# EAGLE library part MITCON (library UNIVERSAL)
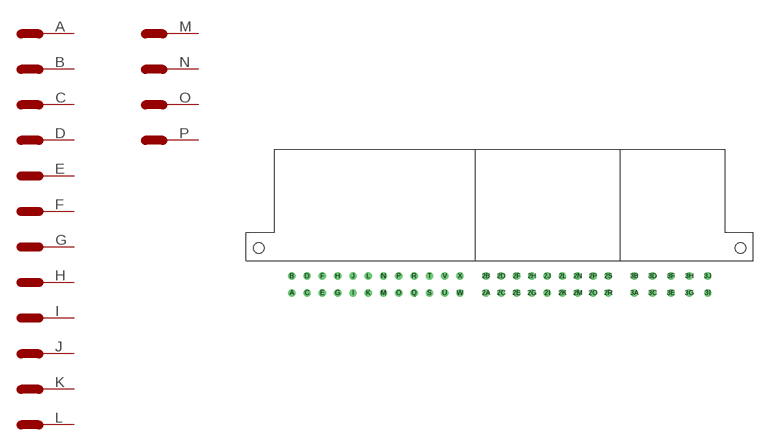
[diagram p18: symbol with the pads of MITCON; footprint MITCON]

Designator prefix CON; gates A=PIN B=PIN C=PIN D=PIN E=PIN F=PIN G=PIN H=PIN I=PIN J=PIN K=PIN L=PIN M=PIN N=PIN O=PIN P=PIN Q=PIN R=PIN S=PIN T=PIN U=PIN V=PIN W=PIN X=PIN 2A=PIN 2B=PIN 2C=PIN 2D=PIN 2E=PIN 2F=PIN 2G=PIN 2H=PIN 2I=PIN 2J=PIN 2K=PIN 2L=PIN 2M=PIN 2N=PIN 2O=PIN 2P=PIN 2R=PIN 2S=PIN 3A=PIN 3B=PIN 3C=PIN 3D=PIN 3E=PIN 3F=PIN 3G=PIN 3H=PIN 3I=PIN 3J=PIN

## MITCON  [MITCON]
2A  2A:1
2B  2B:1
2C  2C:1
2D  2D:1
2E  2E:1
2F  2F:1
2G  2G:1
2H  2H:1
2I  2I:1
2J  2J:1
2K  2K:1
2L  2L:1
2M  2M:1
2N  2N:1
2O  2O:1
2P  2P:1
2R  2R:1
2S  2S:1
3A  3A:1
3B  3B:1
3C  3C:1
3D  3D:1
3E  3E:1
3F  3F:1
3G  3G:1
3H  3H:1
3I  3I:1
3J  3J:1
A  A:1
B  B:1
C  C:1
D  D:1
E  E:1
F  F:1
G  G:1
H  H:1
I  I:1
J  J:1
K  K:1
L  L:1
M  M:1
N  N:1
O  O:1
P  P:1
Q  Q:1
R  R:1
S  S:1
T  T:1
U  U:1
V  V:1
W  W:1
X  X:1

## Footprint MITCON (pad centres in mm)
drill 0.6 pad 1.778: 2A 58.875,-7.875; 2B 58.875,-3.75; 2C 62.625,-7.875; 2D 62.625,-3.75; 2E 66.375,-7.875; 2F 66.375,-3.75; 2G 70.125,-7.875; 2H 70.125,-3.75; 2I 73.875,-7.875; 2J 73.875,-3.75; 2K 77.625,-7.875; 2L 77.625,-3.75; 2M 81.375,-7.875; 2N 81.375,-3.75; 2O 85.125,-7.875; 2P 85.125,-3.75; 2R 88.875,-7.875; 2S 88.875,-3.75; 3A 95.25,-7.875; 3B 95.25,-3.75; 3C 99.75,-7.875; 3D 99.75,-3.75; 3E 104.25,-7.875; 3F 104.25,-3.75; 3G 108.75,-7.875; 3H 108.75,-3.75; 3I 113.25,-7.875; 3J 113.25,-3.75; A 11.25,-7.875; B 11.25,-3.75; C 15,-7.875; D 15,-3.75; E 18.75,-7.875; F 18.75,-3.75; G 22.5,-7.875; H 22.5,-3.75; I 26.25,-7.875; J 26.25,-3.75; K 30,-7.875; L 30,-3.75; M 33.75,-7.875; N 33.75,-3.75; O 37.5,-7.875; P 37.5,-3.75; Q 41.25,-7.875; R 41.25,-3.75; S 45,-7.875; T 45,-3.75; U 48.75,-7.875; V 48.75,-3.75; W 52.5,-7.875; X 52.5,-3.75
